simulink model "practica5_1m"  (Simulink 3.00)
settings: Solver=ode45  StartTime=0.0  StopTime=2  RelTol=1e-3
libraries: cstblocks x1

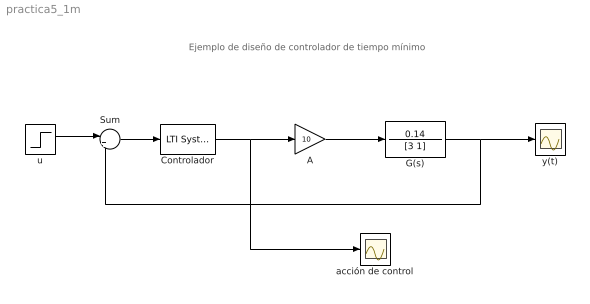
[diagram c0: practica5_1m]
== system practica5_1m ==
  note: Ejemplo de diseño de controlador de tiempo mínimo
  A : Gain  Gain=10  SaturateOnIntegerOverflow=on
  Controlador : cstblocks/LTI System  sys=Dz2  IC=[0]
  G(s) : TransferFcn  Numerator=0.14  Denominator=[3 1]
  Sum : Sum  Inputs=|+-  SaturateOnIntegerOverflow=on
  acción de control : Scope
  u : Step  Time=0  Before=0  After=1  SampleTime=0
  y(t) : Scope
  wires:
  Sum/1 -> Controlador/1
  u/1 -> Sum/1
  G(s)/1 -> Sum/2, y(t)/1
  Controlador/1 -> acción de control/1, A/1
  A/1 -> G(s)/1
